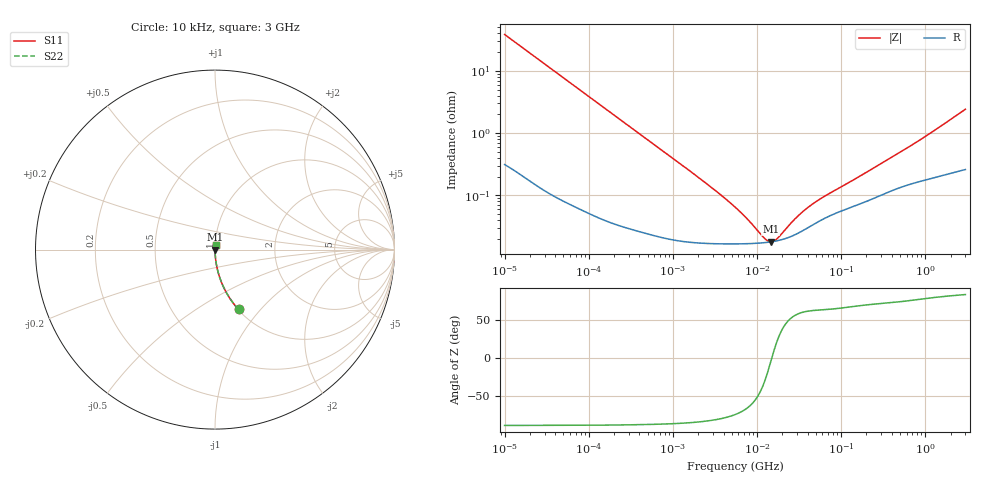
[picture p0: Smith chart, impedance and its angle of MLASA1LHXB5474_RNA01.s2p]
! MLASA1LHXB5474_RNA01  S-PARAMETER MODEL  ( Standard Model )
! Model Generated by TAIYO YUDEN Corporation (http://www.ty-top.com)
! Version 1.0
! TAIYO YUDEN Control No. 220601
! Copyright(c) 2015 TAIYO YUDEN CO.,LTD. All Rights Reserved.
! Product Description (link to TY-COMPAS)
! https://ds.yuden.co.jp/TYCOMPAS/or/detail?pn=MLASA1LHXB5474MRNA01&u=M
! Products Name : Multilayer Ceramic Capacitors
! Characteristics :
!  Capacitance : 0.47 [uF] , Rated Voltage : 4 [V] , TCC : X5R
!  Case Size : 1.0 x 0.5 / 0.039 x 0.02 [mm/inch] , Thickness : 0.13 / 0.005 [mm/inch]
!  (Conditions: Temperature = 25 [degC] , DC Bias Voltage = 0 [V])
! External Node Assignments :
!  1  o---| |---o  2
! GND o---------o GND
! Frequency Range : 10kHz  -  3GHz  [ 401 STEP ]
# MHZ S RI R 50
! Freq[MHz].  S11 Real  S11 Imag  S21 Real  S21 Imag  S12 Real  S12 Imag  S22 Real  S22 Imag
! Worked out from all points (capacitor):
!   401 points, 10 kHz to 3 GHz, reference 50 ohm
!   read as one part in series: C = 413 nF near 10.65 kHz
!   lowest |Z| = 18 mohm at 14.56 MHz (marker M1)
!   series resonance near 15.02 MHz, so ESL is about 270 pH
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0.01  0.1309 -0.3333  0.8691 0.3333  0.8691 0.3333  0.1309 -0.3333
0.016047  0.0564 -0.2264  0.9436 0.2264  0.9436 0.2264  0.0564 -0.2264
0.027426  0.0207 -0.138  0.9793 0.138  0.9793 0.138  0.0207 -0.138
0.045421  0.00808 -0.0846  0.9919 0.0846  0.9919 0.0846  0.00808 -0.0846
0.082683  0.00278 -0.0469  0.9972 0.0469  0.9972 0.0469  0.00278 -0.0469
0.199902  0.00073 -0.0195  0.9993 0.0195  0.9993 0.0195  0.00073 -0.0195
0.683653  0.000249 -0.00576  0.9998 0.00576  0.9998 0.00576  0.000249 -0.00576
2.652321  0.000171 -0.00145  0.9998 0.00145  0.9998 0.00145  0.000171 -0.00145
5.477226  0.000167 -0.000629  0.9998 0.000629  0.9998 0.000629  0.000167 -0.000629
7.747855  0.000168 -0.000376  0.9998 0.000376  0.9998 0.000376  0.000168 -0.000376
12.04705  0.000174 -0.000118  0.9998 0.000118  0.9998 0.000118  0.000174 -0.000118
13.24217  0.000176 -6.67e-05  0.9998 6.67e-05  0.9998 6.67e-05  0.000176 -6.67e-05
14.55585  0.000179 -1.65e-05  0.9998 1.65e-05  0.9998 1.65e-05  0.000179 -1.65e-05
15.99985  0.000183 3.35e-05  0.9998 -3.35e-05  0.9998 -3.35e-05  0.000183 3.35e-05
17.5871  0.000187 8.38e-05  0.9998 -8.38e-05  0.9998 -8.38e-05  0.000187 8.38e-05
29.12589  0.000238 0.000366  0.9998 -0.000366  0.9998 -0.000366  0.000238 0.000366
36.31858  0.000279 0.000499  0.9997 -0.000499  0.9997 -0.000499  0.000279 0.000499
45.28751  0.000332 0.000639  0.9997 -0.000639  0.9997 -0.000639  0.000332 0.000639
64.06182  0.00043 0.000874  0.9996 -0.000874  0.9996 -0.000874  0.00043 0.000874
374.4521  0.00116 0.00372  0.9988 -0.00372  0.9988 -0.00372  0.00116 0.00372
905.3046  0.00176 0.00789  0.9982 -0.00789  0.9982 -0.00789  0.00176 0.00789
3000  0.00317 0.0239  0.9968 -0.0239  0.9968 -0.0239  0.00317 0.0239
